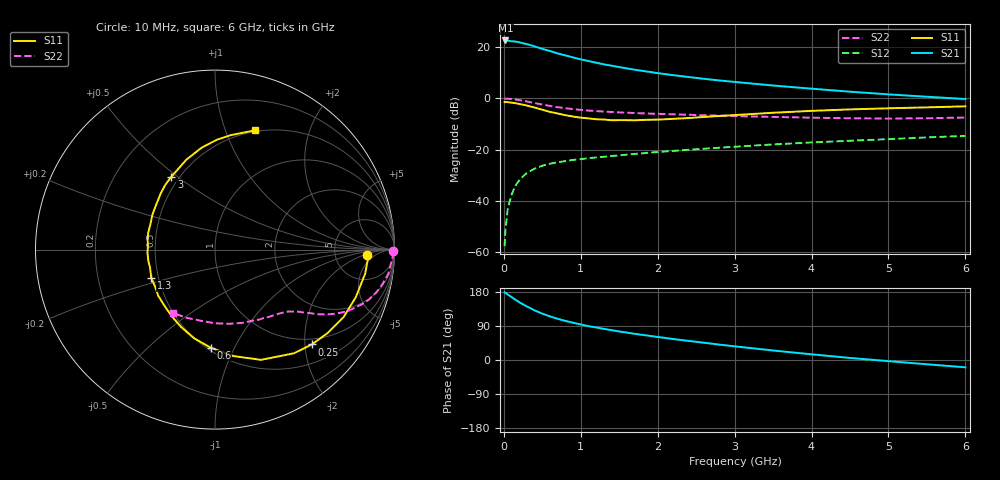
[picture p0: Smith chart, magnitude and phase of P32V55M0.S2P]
! SIEMENS Small Signal Semiconductors
! BFP181
! Si NPN RF Bipolar Junction Transistor in SOT143
! VCE = 2.5 V  IC = 5 mA
! Common Emitter S-Parameters:  March  1996
# GHz  S  MA  R  50
!  f  S11  S21  S12  S22
! GHz  MAG  ANG  MAG  ANG  MAG  ANG  MAG  ANG
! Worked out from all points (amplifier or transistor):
!   36 points, 10 MHz to 6 GHz, reference 50 ohm
!   highest |S21| = 22.7 dB at 20 MHz (marker M1)
!   |S21| within 3 dB of that: start of sweep to 469.9 MHz
!   unconditionally stable (mu >= 1): 1.644 GHz to end of sweep
!   at 250 MHz: K = 0.23, MSG = 26.0 dB, |S12| = -30.4 dB
!   at 1.4 GHz: K = 0.92, MSG = 17.6 dB, |S12| = -22.5 dB
!   at 6 GHz: K = 1.04, MAG = 5.9 dB, |S12| = -14.6 dB
!   lowest NFmin = 1.55 dB at 450 MHz
!   S11 on the Smith chart (normalised r, x): 10 MHz: 12, -2; 250 MHz: 0.87, -2.15; 600 MHz: 0.52, -0.81; 1.3 GHz: 0.46, -0.17; 3 GHz: 0.45, +0.48; 6 GHz: 0.49, +1.28
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0.01  0.8485 -2.0  13.49 178.6  0.0013 81.6  0.9902 -0.6
0.02  0.8528 -3.8  13.6 177.6  0.0026 73.0  0.9925 -1.6
0.05  0.8473 -9.1  13.49 172.9  0.0069 87.8  0.9855 -4.0
0.15  0.8092 -27.7  12.94 159.1  0.0197 74.8  0.9537 -11.5
0.2  0.7816 -36.4  12.52 152.7  0.0252 71.1  0.9294 -14.9
0.25  0.7552 -44.4  11.96 146.6  0.0302 66.4  0.9027 -17.9
0.3  0.7262 -52.7  11.53 141.4  0.035 63.6  0.8726 -20.5
0.4  0.6654 -67.4  10.42 130.9  0.0425 57.4  0.8131 -25.0
0.5  0.6014 -80.3  9.299 122.3  0.0484 52.4  0.7608 -28.0
0.6  0.5471 -92.5  8.441 115.0  0.053 48.9  0.7147 -30.4
0.7  0.5082 -103.1  7.575 108.7  0.0567 46.6  0.6756 -32.2
0.8  0.4708 -113.6  6.946 103.1  0.0597 44.5  0.6451 -33.4
0.9  0.4438 -122.5  6.341 98.4  0.0631 43.1  0.6193 -34.6
1.1  0.408 -140.7  5.394 89.4  0.0683 41.0  0.581 -36.5
1.3  0.3884 -156.1  4.648 82.2  0.0726 39.7  0.5547 -38.5
1.7  0.3739 176.9  3.646 69.2  0.0825 38.8  0.5192 -42.4
2.2  0.3998 150.5  2.856 55.4  0.0945 37.2  0.4898 -48.4
3  0.4734 120.9  2.104 36.1  0.114 33.9  0.4523 -60.3
3.5  0.5256 107.7  1.79 25.1  0.1264 31.2  0.4365 -69.2
4.5  0.6112 89.2  1.356 5.4  0.1492 25.0  0.4105 -90.1
5.5  0.6698 76.5  1.08 -11.3  0.1736 19.4  0.4115 -112.5
6  0.7021 71.3  0.975 -19.3  0.1855 15.7  0.4241 -123.9
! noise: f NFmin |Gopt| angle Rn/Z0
0.45  1.55  0.48  17  0.36
0.9  1.65  0.4  35  0.34
1.8  2  0.18  88  0.34
